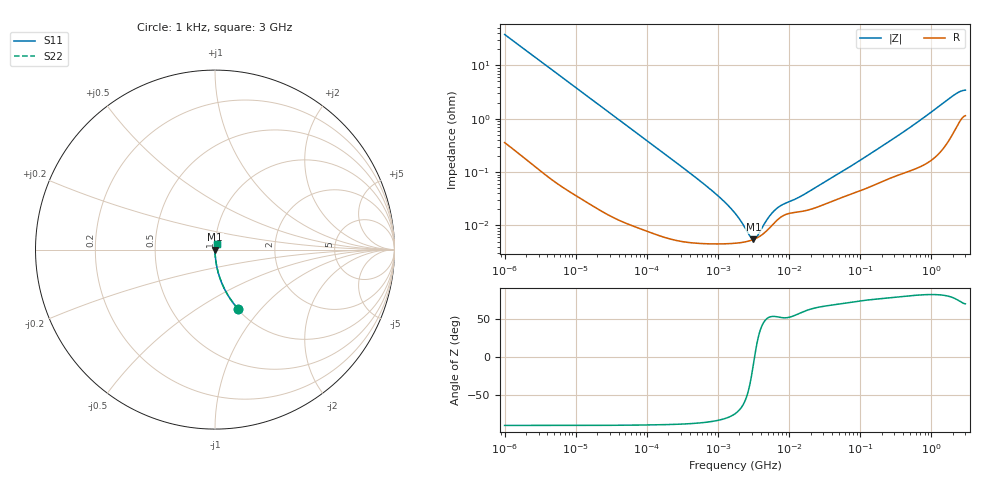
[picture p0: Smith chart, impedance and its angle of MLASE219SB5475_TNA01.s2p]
! MLASE219SB5475_TNA01  S-PARAMETER MODEL  ( Standard Model )
! Model Generated by TAIYO YUDEN Corporation (http://www.ty-top.com)
! Version 1.0
! TAIYO YUDEN Control No. 220601
! Copyright(c) 2009 TAIYO YUDEN CO.,LTD. All Rights Reserved.
! Product Description (link to TY-COMPAS)
! https://ds.yuden.co.jp/TYCOMPAS/or/detail?pn=MLASE219SB5475KTNA01&u=M
! Products Name : Multilayer Ceramic Capacitors
! Characteristics :
!  Capacitance : 4.7 [uF] , Rated Voltage : 16 [V] , TCC : X5R
!  Case Size : 2.0 x 1.25 / 0.079 x 0.049 [mm/inch] , Thickness : 0.85 / 0.033 [mm/inch]
!  (Conditions: Temperature = 25 [degC] , DC Bias Voltage = 0 [V])
! External Node Assignments :
!  1  o---| |---o  2
! GND o---------o GND
! Frequency Range : 1kHz  -  3GHz  [ 401 STEP ]
# MHZ S RI R 50
! Freq[MHz].  S11 Real  S11 Imag  S21 Real  S21 Imag  S12 Real  S12 Imag  S22 Real  S22 Imag
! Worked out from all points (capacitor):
!   401 points, 1 kHz to 3 GHz, reference 50 ohm
!   read as one part in series: C = 4.19 uF near 1.077 kHz
!   lowest |Z| = 5.52 mohm at 3.145 MHz (marker M1)
!   series resonance near 3.255 MHz, so ESL is about 570 pH
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0.001  0.1281 -0.3295  0.8719 0.3295  0.8719 0.3295  0.1281 -0.3295
0.001685  0.0503 -0.214  0.9497 0.214  0.9497 0.214  0.0503 -0.214
0.00306  0.0164 -0.1226  0.9836 0.1226  0.9836 0.1226  0.0164 -0.1226
0.005768  0.00496 -0.066  0.995 0.066  0.995 0.066  0.00496 -0.066
0.01216  0.00131 -0.0316  0.9987 0.0316  0.9987 0.0316  0.00131 -0.0316
0.147855  7.16e-05 -0.00263  0.9999 0.00263  0.9999 0.00263  7.16e-05 -0.00263
0.791611  4.54e-05 -0.000467  1 0.000467  1 0.000467  4.54e-05 -0.000467
1.238299  4.54e-05 -0.000272  1 0.000272  1 0.000272  4.54e-05 -0.000272
1.732051  4.64e-05 -0.000164  1 0.000164  1 0.000164  4.64e-05 -0.000164
2.334012  4.89e-05 -8.28e-05  1 8.28e-05  1 8.28e-05  4.89e-05 -8.28e-05
3.14518  5.45e-05 -8.45e-06  0.9999 8.45e-06  0.9999 8.45e-06  5.45e-05 -8.45e-06
4.238263  6.84e-05 6.54e-05  0.9999 -6.54e-05  0.9999 -6.54e-05  6.84e-05 6.54e-05
5.928204  0.000105 0.000145  0.9999 -0.000145  0.9999 -0.000145  0.000105 0.000145
7.143107  0.000134 0.000178  0.9999 -0.000178  0.9999 -0.000178  0.000134 0.000178
13.97519  0.000181 0.00029  0.9998 -0.00029  0.9998 -0.00029  0.000181 0.00029
21.06097  0.000205 0.000424  0.9998 -0.000424  0.9998 -0.000424  0.000205 0.000424
80.61565  0.000403 0.00133  0.9996 -0.00133  0.9996 -0.00133  0.000403 0.00133
256.0921  0.00077 0.00369  0.9992 -0.00369  0.9992 -0.00369  0.00077 0.00369
626.6478  0.00125 0.00841  0.9987 -0.00841  0.9987 -0.00841  0.00125 0.00841
2066.299  0.00633 0.0268  0.9937 -0.0268  0.9937 -0.0268  0.00633 0.0268
2489.759  0.00965 0.0303  0.9903 -0.0303  0.9903 -0.0303  0.00965 0.0303
3000  0.0123 0.0317  0.9877 -0.0317  0.9877 -0.0317  0.0123 0.0317
